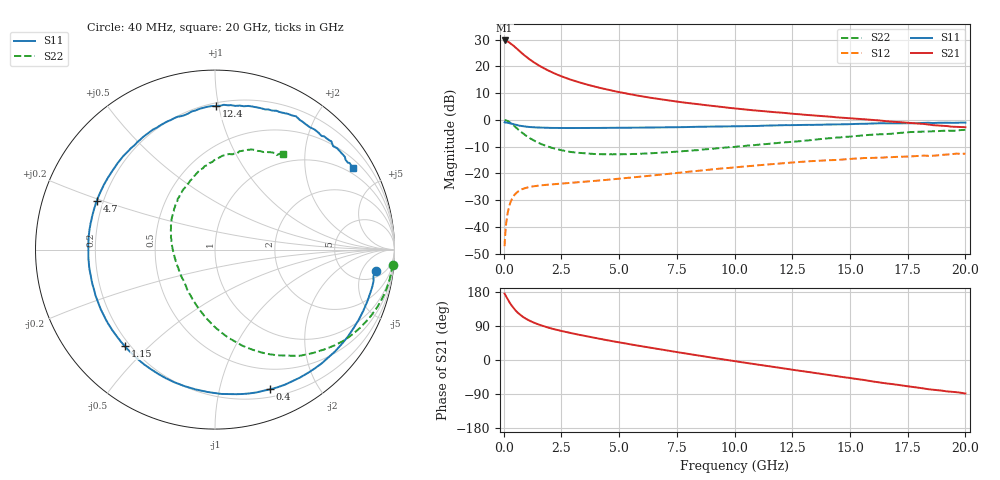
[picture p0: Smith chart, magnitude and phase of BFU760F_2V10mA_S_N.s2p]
! Filename:  P:\Prog\Test\Noise\ATS_data\Testdata_Net\BFU760\BFU760F_2W_C1_2V10mA_D.s2p
! Date/Time: Mon 06/Feb/2012 15:05:22
! BFU760_2W_C1_2V10mA
! bias mode 1: Vout= 2.0001 V, Iout=10.0600 mA, Vin= 0.7726 V, Iin= 0.0293 mA
! Date/time Fri Mar 18 10:03:34 2011
! Device data file deembeded for feedlines and parallel
! Original file: \BFU760\BFU760_2W_C1_2V10mA_R.s2p
! Feed-files: PR003V01_101208_Feed1.s2p, PR003V01_101208_Feed2.s2p
! Parallel-file: PR003V01_101208_Par.s2p
# MHz S MA R 50
!  Freq-MHz  S11-mag  S11-arg  S21-mag  S21-arg  S12-mag  S12-arg  S22-mag  S22-arg
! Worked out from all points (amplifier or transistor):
!   167 points, 40 MHz to 20 GHz, reference 50 ohm
!   highest |S21| = 29.7 dB at 40 MHz (marker M1)
!   |S21| within 3 dB of that: start of sweep to 560.5 MHz
!   unconditionally stable (mu >= 1): 5.216 GHz to 13.51 GHz
!   at 550 MHz: K = 0.13, MSG = 27.0 dB, |S12| = -27.3 dB
!   at 4.2 GHz: K = 0.89, MSG = 17.3 dB, |S12| = -22.6 dB
!   at 20 GHz: K = 0.84, MSG = 5.0 dB, |S12| = -12.6 dB
!   lowest NFmin = 0.46 dB at 800 MHz
!   S11 on the Smith chart (normalised r, x): 40 MHz: 7, -9; 400 MHz: 0.28, -1.43; 1.15 GHz: 0.18, -0.42; 4.7 GHz: 0.17, +0.19; 12.4 GHz: 0.22, +0.98; 20 GHz: 0.78, +3.49
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40  0.9021 -7.5  30.6 175.4  0.004373 84.6  0.9931 -4.8
50  0.8947 -9.7  30.59 173.7  0.005611 79.1  0.9917 -6.1
140  0.8913 -26.0  29.66 163.9  0.01495 76.5  0.9681 -17.1
240  0.8715 -43.7  28.12 153.3  0.02439 67.8  0.9172 -28.5
320  0.8558 -56.4  26.43 146.0  0.03073 61.4  0.8658 -37.0
400  0.8367 -68.5  24.94 139.2  0.03605 56.0  0.8096 -44.3
550  0.805 -87.5  21.88 128.5  0.0433 47.5  0.709 -56.4
650  0.7864 -97.9  19.94 122.7  0.04689 43.0  0.6519 -63.1
750  0.7732 -107.0  18.29 117.6  0.04961 39.5  0.5997 -69.0
950  0.7518 -121.7  15.47 109.4  0.05354 34.2  0.5152 -78.8
1150  0.7366 -133.0  13.31 102.9  0.05613 30.5  0.452 -87.1
1500  0.722 -147.6  10.59 94.0  0.05909 26.4  0.375 -99.0
1950  0.7106 -160.8  8.318 85.1  0.06177 23.6  0.315 -111.3
2500  0.7076 -172.5  6.544 76.6  0.06448 22.2  0.2728 -124.3
3400  0.7073 173.4  4.864 64.9  0.06931 21.3  0.2406 -140.7
4700  0.7125 157.5  3.531 49.8  0.0776 21.1  0.2277 -161.6
6800  0.727 136.4  2.434 27.9  0.09498 18.8  0.2442 171.7
10200  0.7668 107.2  1.612 -4.8  0.1321 8.0  0.3215 135.2
12400  0.799 89.4  1.325 -24.6  0.159 -2.6  0.3875 114.7
13400  0.8086 82.0  1.215 -33.4  0.1706 -9.0  0.4241 106.1
16800  0.8633 55.5  0.9293 -63.4  0.2015 -29.7  0.5522 76.9
20000  0.8926 30.6  0.7319 -88.3  0.2337 -51.6  0.6523 54.7
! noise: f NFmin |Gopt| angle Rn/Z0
400  0.4577  0.1687  17.23  0.0628
700  0.4552  0.1696  47.66  0.0621
1100  0.4567  0.2037  77.09  0.0602
1500  0.4639  0.2452  96.61  0.0572
1900  0.4766  0.2836  111.7  0.0535
2350  0.4976  0.3229  126.2  0.0489
3000  0.5405  0.378  144.9  0.0422
3800  0.6135  0.4481  164.4  0.0356
4600  0.7089  0.5106  180.1  0.0329
6000  0.9297  0.5235  201.2  0.0448
